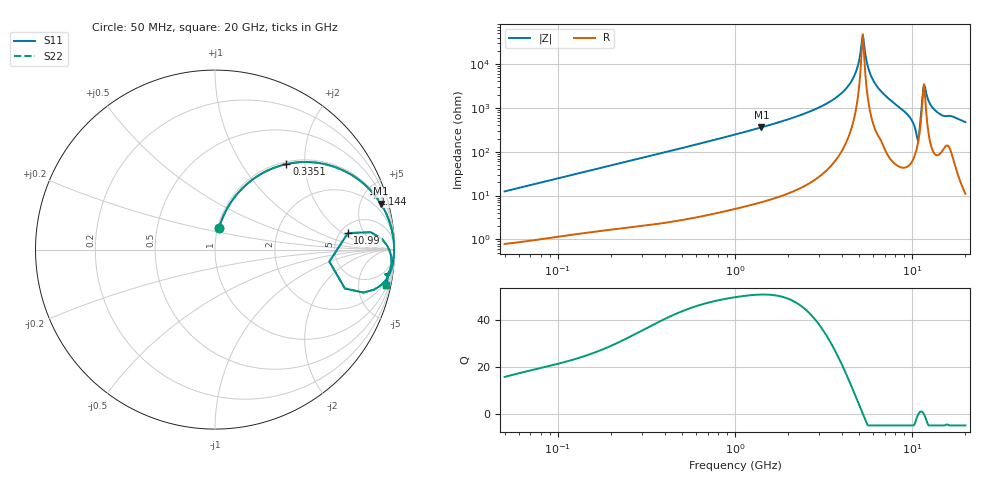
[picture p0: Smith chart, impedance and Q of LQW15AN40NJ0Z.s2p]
!Murata Part Number: LQW15AN40NJ0Z
!These Parameters are Measured in Series Mode Connection
!  o--[Z]--o
!Port1  Port2
!  o-------o
!Freq. Start=50[MHz] Stop=20[GHz], 401[Steps]
# Hz S RI R 50
!Freq.(Hz) S11(Real) S11(Imag) S21(Real) S21(Imag) S12(Real) S12(Imag) S22(Real) S22(Imag)
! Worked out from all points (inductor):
!   401 points, 50 MHz to 20 GHz, reference 50 ohm
!   read as one part in series: L = 39.4 nH near 51.52 MHz
!   highest Q = 51 at 1.411 GHz (marker M1), where L = 40.5 nH
!   self-resonance near 5.195 GHz
!   S11 on the Smith chart (normalised r, x): 50 MHz: 1.02, +0.25; 335.1 MHz: 1.04, +1.62; 1.144 GHz: 1.11, +5.69; 10.99 GHz: 5.84, +2.42; 20 GHz: 1.22, -9.48
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5e7  0.0227 0.1205  0.9773 -0.1205  0.9773 -0.1205  0.0227 0.1205
1.364002e8  0.1095 0.2924  0.8905 -0.2924  0.8905 -0.2924  0.1095 0.2924
3.350611e8  0.398 0.4764  0.602 -0.4764  0.602 -0.4764  0.398 0.4764
3.721004e8  0.4477 0.4847  0.5523 -0.4847  0.5523 -0.4847  0.4477 0.4847
1e9  0.8537 0.3435  0.1463 -0.3435  0.1463 -0.3435  0.8537 0.3435
1.144317e9  0.8855 0.3087  0.1145 -0.3087  0.1145 -0.3087  0.8855 0.3087
1.411297e9  0.9239 0.2555  0.0761 -0.2555  0.0761 -0.2555  0.9239 0.2555
2.728004e9  0.9844 0.1127  0.0156 -0.1127  0.0156 -0.1127  0.9844 0.1127
4.34015e9  0.9969 0.0322  0.00314 -0.0322  0.00314 -0.0322  0.9969 0.0322
4.81993e9  0.9977 0.0148  0.0023 -0.0148  0.0023 -0.0148  0.9977 0.0148
5.273168e9  0.9979 -0.000162  0.00211 0.000162  0.00211 0.000162  0.9979 -0.000162
5.944466e9  0.9973 -0.0208  0.00275 0.0208  0.00275 0.0208  0.9973 -0.0208
7.442007e9  0.9931 -0.063  0.00694 0.063  0.00694 0.063  0.9931 -0.063
9.457416e9  0.9707 -0.1385  0.0293 0.1385  0.0293 0.1385  0.9707 -0.1385
1.034674e10  0.8868 -0.2228  0.1132 0.2228  0.1132 0.2228  0.8868 -0.2228
1.066139e10  0.7238 -0.2167  0.2762 0.2167  0.2762 0.2167  0.7238 -0.2167
1.098561e10  0.74 0.0919  0.26 -0.0919  0.26 -0.0919  0.74 0.0919
1.149051e10  0.9591 0.0225  0.0409 -0.0225  0.0409 -0.0225  0.9591 0.0225
1.183995e10  0.9785 -0.0251  0.0215 0.0251  0.0215 0.0251  0.9785 -0.0251
1.276073e10  0.9821 -0.0839  0.0179 0.0839  0.0179 0.0839  0.9821 -0.0839
1.396067e10  0.9711 -0.1221  0.0289 0.1221  0.0289 0.1221  0.9711 -0.1221
2e10  0.9531 -0.2  0.0469 0.2  0.0469 0.2  0.9531 -0.2
